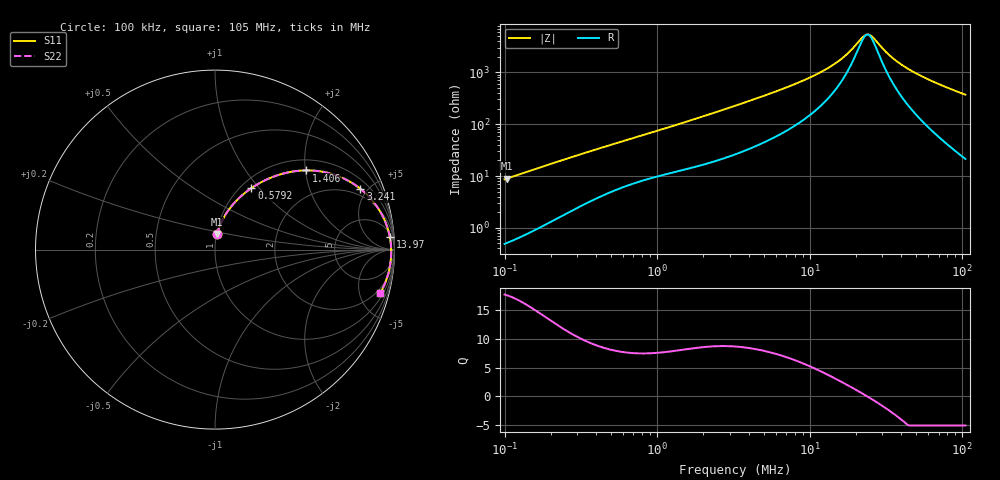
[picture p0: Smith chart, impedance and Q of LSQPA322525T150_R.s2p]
! LSQPA322525T150_R  S-PARAMETER MODEL  ( General Type )
! Model Generated by TAIYO YUDEN Corporation (http://www.ty-top.com)
! Version 2.0
! TAIYO YUDEN Control No. 100810NF25SB-FAC
! Copyright(c) 2007 TAIYO YUDEN CO.,LTD. All Rights Reserved.
! Product Description (link to TY-COMPAS)
! https://ds.yuden.co.jp/TYCOMPAS/or/detail?pn=LSQPA322525T150KR&u=M
! Products Name : Inductors
! Characteristics :
!  Inductance : 15 uH , SRF(min) : 20 MHz , DC Resistance(max) : 0.2535 Ohm
!  Rated Current : Saturation :730 mA , Temp Rise : 850 mA (40 degC)
!  Case Size : 3.2 x 2.5 / 0.126 x 0.098 [mm/inch] , Thickness : 2.5 / 0.098 [mm/inch]
!  (Conditions: Temperature = 25 degC , DC Bias Current/Voltage = 0A / 0V)
! External Node Assignments :
!  1  o---GGG---o  2
! GND o---------o GND
! Frequency Range : 0.1MHz  -  105.0131MHz  [ 402 STEP ]
# MHz S RI R 50
! Freq[MHz].  S11 Real  S11 Imag  S21 Real  S21 Imag  S12 Real  S12 Imag  S22 Real  S22 Imag
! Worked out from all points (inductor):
!   401 points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, 100 kHz to 105 MHz, reference 50 ohm
!   read as one part in series: L = 13.7 uH near 103.5 kHz
!   highest Q = 17.5 at 103.5 kHz (marker M1), where L = 13.7 uH
!   self-resonance near 23.93 MHz
!   S11 on the Smith chart (normalised r, x): 100 kHz: 1.01, +0.17; 579.2 kHz: 1.12, +0.91; 1.406 MHz: 1.25, +2.02; 3.241 MHz: 1.52, +4.50; 13.97 MHz: 9, +26; 105 MHz: 1.43, -7.41
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0.1  0.0122 0.0848  0.9878 -0.0848  0.9878 -0.0848  0.0122 0.0848
0.10354  0.0129 0.0877  0.9871 -0.0877  0.9871 -0.0877  0.0129 0.0877
0.19365  0.0377 0.1567  0.9623 -0.1567  0.9623 -0.1567  0.0377 0.1567
0.32067  0.0874 0.2365  0.9126 -0.2365  0.9126 -0.2365  0.0874 0.2365
0.579247  0.2024 0.3422  0.7976 -0.3422  0.7976 -0.3422  0.2024 0.3422
1.028292  0.3832 0.4245  0.6168 -0.4245  0.6168 -0.4245  0.3832 0.4245
1.406282  0.5075 0.4413  0.4925 -0.4413  0.4925 -0.4413  0.5075 0.4413
2.061773  0.6627 0.418  0.3373 -0.418  0.3373 -0.418  0.6627 0.418
3.240572  0.8106 0.3382  0.1894 -0.3382  0.1894 -0.3382  0.8106 0.3382
3.297424  0.8151 0.3345  0.1849 -0.3345  0.1849 -0.3345  0.8151 0.3345
6.275378  0.9279 0.1985  0.0721 -0.1985  0.0721 -0.1985  0.9279 0.1985
10.39154  0.9644 0.1108  0.0356 -0.1108  0.0356 -0.1108  0.9644 0.1108
13.96635  0.9746 0.0683  0.0254 -0.0683  0.0254 -0.0683  0.9746 0.0683
17.2076  0.9788 0.0409  0.0212 -0.0409  0.0212 -0.0409  0.9788 0.0409
21.95147  0.9814 0.0106  0.0186 -0.0106  0.0186 -0.0106  0.9814 0.0106
23.53294  0.9817 0.00206  0.0183 -0.00206  0.0183 -0.00206  0.9817 0.00206
25.67093  0.9819 -0.00864  0.0181 0.00864  0.0181 0.00864  0.9819 -0.00864
33.32256  0.9809 -0.0416  0.0191 0.0416  0.0191 0.0416  0.9809 -0.0416
40.34804  0.9785 -0.0674  0.0215 0.0674  0.0215 0.0674  0.9785 -0.0674
52.37441  0.972 -0.1065  0.028 0.1065  0.028 0.1065  0.972 -0.1065
72.88333  0.9558 -0.1649  0.0442 0.1649  0.0442 0.1649  0.9558 -0.1649
105.0131  0.9201 -0.2439  0.0799 0.2439  0.0799 0.2439  0.9201 -0.2439
